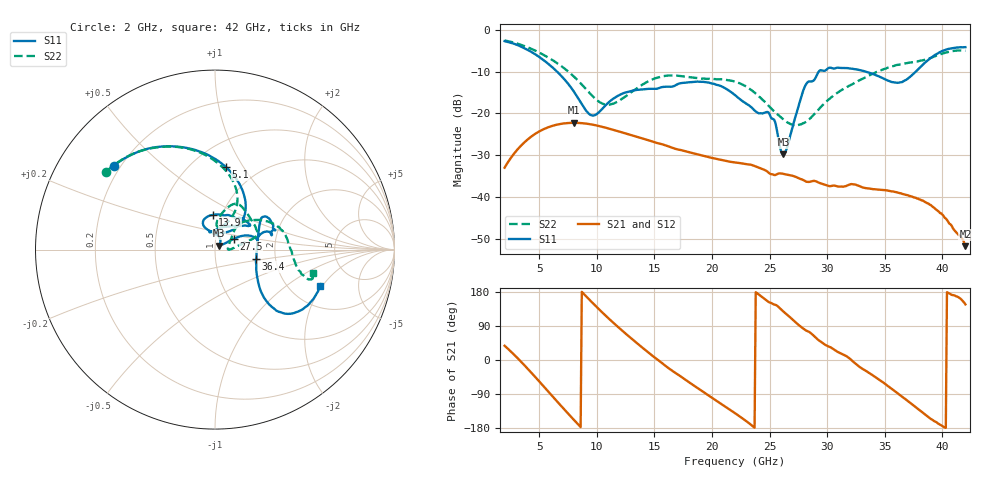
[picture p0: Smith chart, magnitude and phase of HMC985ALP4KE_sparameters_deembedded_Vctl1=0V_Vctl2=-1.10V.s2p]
!s2p File: Measurements: S11, S21, S12, S22
# GHz S dB R 50.0
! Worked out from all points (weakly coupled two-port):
!   401 points, 2 GHz to 42 GHz, reference 50 ohm
!   highest |S21| = -22.24 dB at 8 GHz (marker M1); lowest = -51.8 dB at 42 GHz (marker M2)
!   lowest |S11| = -29.8 dB at 26.2 GHz (marker M3), VSWR 1.07, Z = 52.4 + j2.27 ohm
!   |S11| at or under -10 dB: 6.553 GHz to 29.27 GHz (22.72 GHz wide, 127 % of centre); 33.35 GHz to 37.69 GHz (4.344 GHz wide, 12.2 % of centre)
!   |S22| runs from -22.9 to -2.5 dB; largest |S21 - S12| = 0.00017
!   S11 on the Smith chart (normalised r, x): 2 GHz: 0.17, +0.35; 5.1 GHz: 0.72, +0.84; 13.9 GHz: 0.90, +0.36; 27.5 GHz: 1.22, +0.15; 36.4 GHz: 1.58, -0.18; 42 GHz: 2.90, -1.91
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2  -2.70 140.3  -32.98 37.6  -32.99 37.7  -2.54 144.4
3.5  -4.11 112.6  -27.51 -6.8  -27.51 -6.8  -3.66 119.8
5.1  -6.68 82.5  -24.17 -59.7  -24.17 -59.8  -5.57 95.3
8  -14.72 45.7  -22.25 -157.5  -22.25 -157.6  -11.14 63.8
8.7  -17.79 51.8  -22.33 179.9  -22.33 179.9  -13.09 62.3
9.7  -20.52 85.5  -22.72 148.7  -22.72 148.7  -16.04 67.1
10.9  -17.70 113.6  -23.52 113.3  -23.52 113.3  -17.91 81.1
13.9  -14.25 93.9  -25.94 34.1  -25.94 34.0  -13.21 77.3
15.4  -13.94 73.0  -27.18 -1.8  -27.18 -1.8  -11.32 68.4
19.4  -12.52 34.6  -30.25 -87.3  -30.26 -87.4  -11.70 36.4
22  -15.61 52.3  -31.73 -140.3  -31.73 -140.3  -12.41 17.9
25  -20.18 97.9  -34.37 151.8  -34.37 151.8  -18.41 8.0
26.2  -29.81 42.0  -34.46 127.9  -34.46 127.9  -21.47 0.5
27.5  -18.40 29.8  -35.46 92.9  -35.47 93.0  -22.76 5.8
28.1  -13.36 20.7  -36.20 79.2  -36.21 78.9  -22.12 16.0
28.7  -12.31 12.9  -36.20 67.9  -36.21 67.9  -20.70 26.4
31  -9.08 23.3  -37.51 20.1  -37.50 20.2  -14.83 46.9
33.3  -9.96 34.4  -37.85 -27.7  -37.86 -27.6  -11.41 37.6
35.4  -12.27 12.3  -38.55 -71.6  -38.55 -71.6  -8.96 23.7
36.4  -12.57 -12.8  -39.12 -94.4  -39.16 -94.5  -8.19 15.9
39.5  -5.81 -43.3  -43.09 -164.3  -43.07 -165.7  -6.17 -14.5
42  -4.14 -19.0  -51.77 146.8  -51.47 146.4  -5.01 -13.2
